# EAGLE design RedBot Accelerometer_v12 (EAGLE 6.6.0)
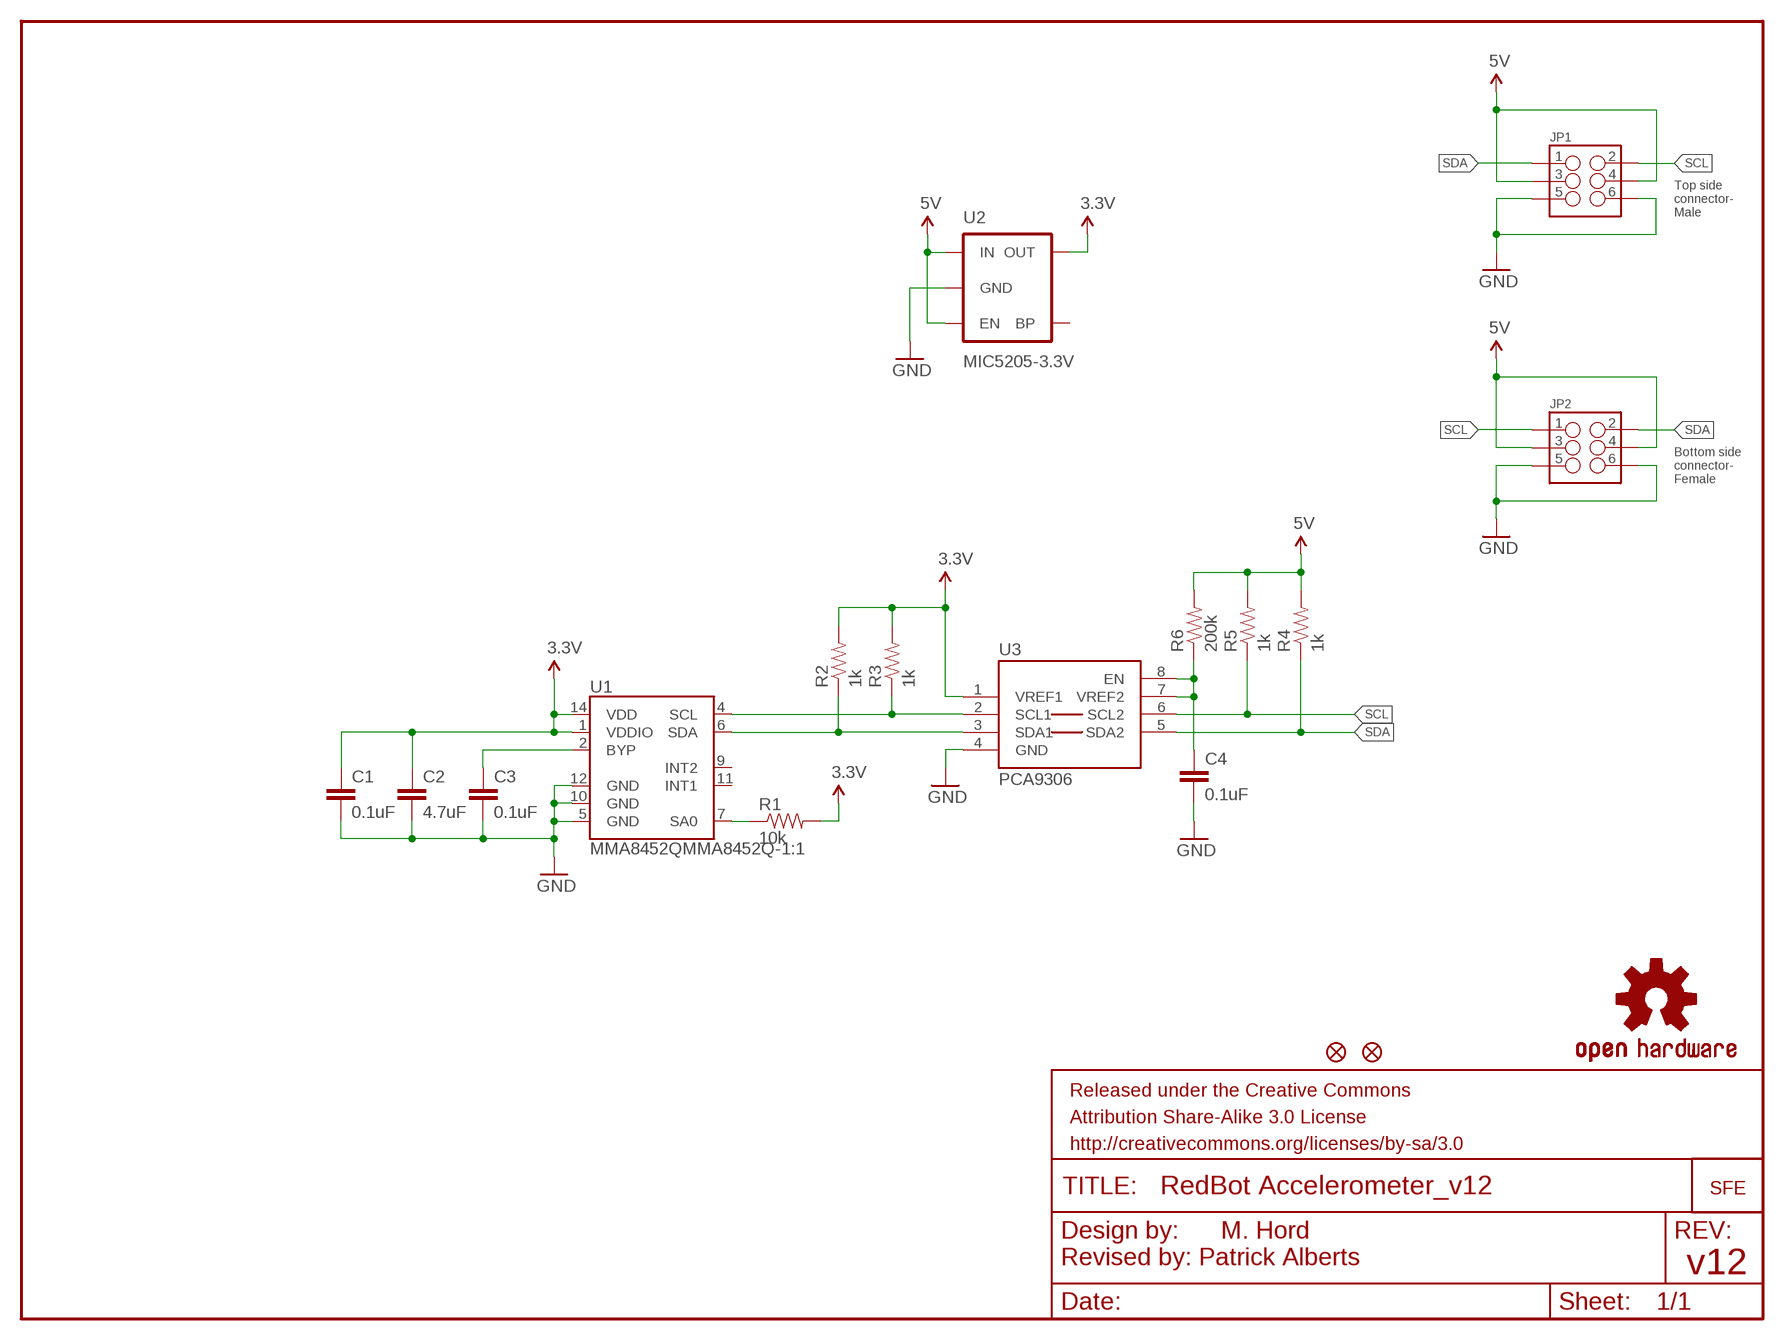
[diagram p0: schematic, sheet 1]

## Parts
C1  0.1uF  0.1UF-25V(+80/-20%)(0603)  [0603-CAP]
C2  4.7uF  4.7UF-6.3V-10%(0603)0603  [0603-CAP]
C3  0.1uF  0.1UF-25V(+80/-20%)(0603)  [0603-CAP]
C4  0.1uF  0.1UF-25V(+80/-20%)(0603)  [0603-CAP]
FID1  FIDUCIAL1X2  [FIDUCIAL-1X2]
FID3  FIDUCIAL1X2  [FIDUCIAL-1X2]
FRAME1  FRAME-LETTER  [CREATIVE_COMMONS]
JP1  M03X2SMT  [2X3_SMT_POSTS]
JP2  M03X2FEMALE_SMD  [2X3_SMD]
LOGO1  LOGO-SFESK  [SFE-LOGO-FLAME]
LOGO2  OSHW-LOGOS  [OSHW-LOGO-S]
R1  10k  10KOHM1/10W1%(0603)0603  [0603-RES]
R2  1k  1K-1%  [0603-RES]
R3  1k  1K-1%  [0603-RES]
R4  1k  1K-1%  [0603-RES]
R5  1k  1K-1%  [0603-RES]
R6  200k  200KOHM1/10W1%(0603)200K  [0603-RES]
U1  MMA8452QMMA8452Q-1:1  [MMA8452Q-1:1]
U2  MIC5205-3.3V  MIC52053.3V  [SOT23-5]
U3  PCA9306  PCA9306PCA9306DC-1:1  [PCA9306DC-1:1]

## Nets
3.3V: C1.1 C2.1 R1.2 R2.2 R3.2 U1.1(VDDIO) U1.14(VDD) U2.5(OUT) U3.1(VREF1)
5V: JP1.3 JP1.4 JP2.3 JP2.4 R4.2 R5.2 R6.2 U2.1(IN) U2.3(EN)
ADDR: R1.1 U1.7(SA0)
GND: C1.2 C2.2 C3.2 C4.2 JP1.5 JP1.6 JP2.5 JP2.6 U1.5(GND) U1.10(GND) U1.12(GND) U2.2(GND) U3.4(GND)
N$1: C3.1 U1.2(BYP)
N$2: C4.1 R6.1 U3.7(VREF2) U3.8(EN)
SCL: JP1.2 JP2.1 R5.1 U3.6(SCL2)
SCL1: R3.1 U1.4(SCL) U3.2(SCL1)
SDA: JP1.1 JP2.2 R4.1 U3.5(SDA2)
SDA1: R2.1 U1.6(SDA) U3.3(SDA1)
Unconnected: U1.9(INT2) U1.11(INT1) U2.4(BP)

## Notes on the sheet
- Top side
  connector-
  Male
- Bottom side
  connector-
  Female
- M. Hord
- Revised by: Patrick Alberts
- v12

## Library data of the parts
C1 C3 C4 = SparkFun-Capacitors:0.1UF-25V(+80/-20%)(0603): Ceramic; PROD_ID: CAP-00810
C2 = SparkFun-Capacitors:4.7UF-6.3V-10%(0603): CAP-08280; PROD_ID: CAP-08280
FID1 FID3 = SparkFun-Aesthetics:FIDUCIAL: Fiducial Alignment Points
FRAME1 = SparkFun-Aesthetics:FRAME-LETTER: Schematic Frame
JP1 = SparkFun-Connectors:M03X2: 2x3 .1" header. Shrouded, with keying- CONN-10681 SMT- CONN-11415 Pogo pins- HW-11044; PROD_ID: CONN-11415
JP2 = SparkFun-Connectors:M03X2: 2x3 .1" header. Shrouded, with keying- CONN-10681 SMT- CONN-11415 Pogo pins- HW-11044; PROD_ID: CONN-11290
LOGO1 = SparkFun-Aesthetics:LOGO-SFE: Spark Fun Electronics PCB Logo
LOGO2 = SparkFun-Aesthetics:OSHW-LOGO: Open Source Hardware Logo This logo indicates the piece of hardware it is found on incorporates a OSHW license and/or adheres to the definition of open source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
R1 = SparkFun-Resistors:10KOHM1/10W1%(0603): RES-00824; PROD_ID: RES-00824; VALUE: 10K
R2-R5 = SparkFun-Resistors:1K-1%: 1k-ohm SMT; PROD_ID: RES-07856
R6 = SparkFun-Resistors:200KOHM1/10W1%(0603): RES-09385; PROD_ID: RES-09385
U1 = SparkFun-Sensors:MMA8452Q: MMA8452Q 3-Axis, 12/8-bit Digital Accelerometer Supply Voltage: 1.6-3.6V Range: +/- 2g, 4g, 8g Interface: I2C, 12-bit and 8-bit ODR: 1.56 Hz - 800 Hz Package: QFN-16 http://cache.freescale.com/files/sensors/doc/data_sheet/MMA8452Q.pdf
U2 = SparkFun-PowerIC:MIC5205: MIC5205 150mA vreg 3.3V - VREG-00822 5V - VREG-00823; PROD_ID: VREG-00822
U3 = SparkFun-DigitalIC:PCA9306: Bidirectional I2C level shifter. NOT compatible with all available part number pinout schemes- DOUBLE CHECK!!!

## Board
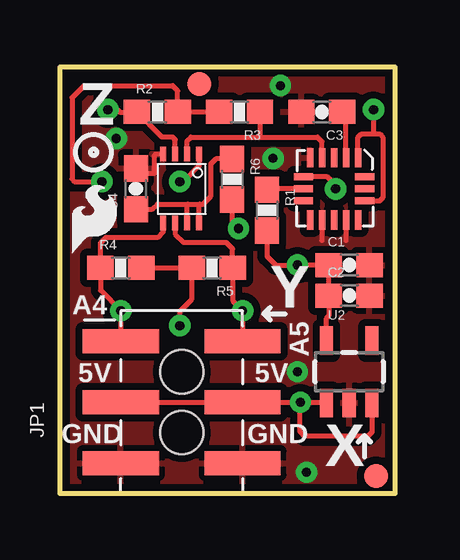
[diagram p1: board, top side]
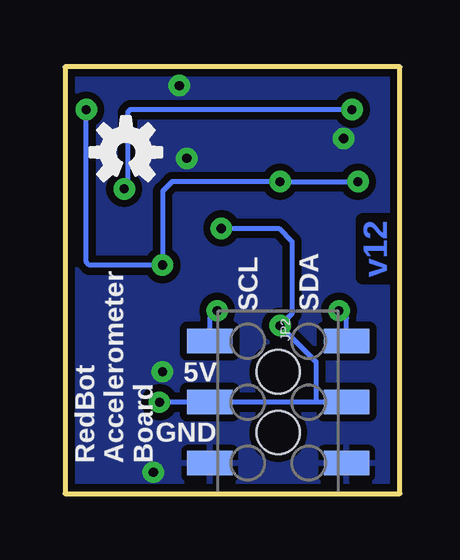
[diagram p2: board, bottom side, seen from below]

Size 13.97 x 17.78 mm. Coordinates in mm from the lower left corner, seen from the top.
Outline: 0,0 0,17.78 13.97,17.78 13.97,0 0,0
Copper layers (1*16): Top 0.035mm / dielectric 1.5mm / Bottom 0.035mm
Design rules "SparkFun-2-layer": minimum track width 7mil, minimum drill 15mil, track to track 8mil, track to pad 8mil, pad to pad 8mil, via to via 8mil, smd to smd 8mil, copper to edge 8mil, drill to drill 8mil, minimum pad ring 12mil, minimum via ring 10mil, stop-mask expansion 4mil, vias tented up to drill 20mil, thermal gap 10mil

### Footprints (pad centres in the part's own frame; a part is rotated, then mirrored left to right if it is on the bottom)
0603-CAP = smd 1.1 x 1: 1 -0.85,0; 2 0.85,0
FIDUCIAL-1X2 = smd 1 x 1: 1 0,0
2X3_SMT_POSTS = smd 1 x 3.17: 1 -2.54,-2.54; 2 -2.54,2.54; 3 0,-2.54; 4 0,2.54; 5 2.54,-2.54; 6 2.54,2.54 | hole 1.8: -1.27,0; 1.27,0
2X3_SMD = smd 1.02 x 1.9: 1 -2.54,-2.85; 2 -2.54,2.85; 3 0,-2.85; 4 0,2.85; 5 2.54,-2.85; 6 2.54,2.85
0603-RES = smd 1.1 x 1: 1 -0.85,0; 2 0.85,0
MMA8452Q-1:1 = smd 0.8 x 0.275: 1 -1.3,1; 2 -1.3,0.5; 3 -1.3,0; 4 -1.3,-0.5; 5 -1.3,-1; 9 1.3,-1; 10 1.3,-0.5; 11 1.3,0; 12 1.3,0.5; 13 1.3,1 | smd 0.29 x 0.8: 6 -0.5,-1.275; 7 0,-1.275; 8 0.5,-1.275; 14 0.5,1.275; 15 0,1.275; 16 -0.5,1.275
SOT23-5 = smd 0.55 x 1.2: 1 -0.95,-1.3; 2 0,-1.3; 3 0.95,-1.3; 4 0.95,1.3; 5 -0.95,1.3
PCA9306DC-1:1 = smd 0.25 x 0.602: 1 -0.73,-1.446; 2 -0.23,-1.446; 3 0.27,-1.446; 4 0.77,-1.446; 5 0.77,1.431; 6 0.27,1.431; 7 -0.23,1.431; 8 -0.73,1.431

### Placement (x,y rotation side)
C1  12.06,9.53 0 top
C2  12.06,8.26 0 top
C3  10.92,15.9 180 top
C4  3.17,12.7 90 top
FID1  5.82,17.07 0 top
FID3  13.18,0.74 0 top
FRAME1  not placed on the board
JP1  5.08,3.81 270 top
JP2  5.08,3.81 270 bottom
LOGO1  0.51,10.03 0 top
LOGO2  11.43,14.22 0 bottom
R1  8.64,11.81 270 top
R2  4.06,15.9 0 top
R3  7.49,15.9 180 top
R4  2.54,9.4 0 top
R5  6.35,9.4 180 top
R6  7.18,13.1 270 top
U1  11.43,12.7 270 top
U2  12.06,5.08 0 top
U3  5.08,12.7 180 top

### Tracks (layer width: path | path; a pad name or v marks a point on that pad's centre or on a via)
3.3V  (via drill 0.38)
  Top 0.203: U2.5 11.12,7.3 11.21,7.41 C2.1 C1.1 v9.91,9.53 9,9.53 8.64,9.89 R1.2 | R3.2 R2.2 4.91,16.79 4.7,17 1,17 0.5,16.5 0.5,13.1 0.6,13 v1.75,13 | U1.1 12.43,14.84 12.57,14.99 13.08,14.99 | 13.08,14.99 13.34,14.99 13.46,14.86 13.46,12.32 13.34,12.2 U1.14 | v13.08,16 13.08,14.99 | v5,13 5.15,13 5.81,13.66 U3.1
  Bottom 0.203: v13.08,16 13.08,9.65 12.95,9.53 v9.91,9.53 v9.9,9.53 9.9,12.6 9.5,13 v5,13 v1.75,13
5V  (via drill 0.38)
  Top 0.203: v10.03,3.81 JP1.4 JP1.3 | v10.03,3.81 11.09,3.81 U2.1 | R4.2 R5.2 5.5,8.1 5,7.6 v5,7 | U2.3 13.02,2.56 12.85,2.4 10.2,2.4 10,2.6 10,3.78 v10.03,3.81 | R6.2 7.18,11.31 v7.45,11.05
  Bottom 0.203: v10.03,3.81 JP2.3 3.5,3.81 | JP2.4 3.5,3.81 | v7.45,11.05 5.05,11.05 4.5,10.5 4.5,7.5 v5,7 3.5,5.5 3.5,3.81
ADDR
  Top 0.203: U1.7 8.68,12.7 R1.1
GND  (via drill 0.38)
  Top 0.203: U1.12 11.93,10.55 11.94,10.54 | U1.10 10.93,10.55 10.92,10.54 | U3.4 3.99,14.15 3.94,14.1 3.94,13.34 3.39,13.34 C4.2
  other vias: 10.29,0.89 9.91,5.08 8.89,13.97 9.2,17 2.35,14.8
  pour Top (isolate 0.305): 0,17.78 13.97,17.78 13.97,0 0,0
  pour Bottom (isolate 0.305): 0,17.78 13.97,17.78 13.97,0 0,0
N$1
  Top 0.203: U1.2 11.93,15.74 C3.1
N$2
  Top 0.203: C4.1 3.85,11.85 4.06,12.06 5.33,12.06 | 5.33,12.06 5.84,12.06 | 5.84,12.06 5.97,12.06 6.3,12.39 6.3,13.75 6.5,13.95 R6.1 | U3.8 5.81,12.03 5.84,12.06 | U3.7 5.31,12.04 5.33,12.06
SCL  (via drill 0.38)
  Top 0.203: U3.6 4.81,10.81 5.15,10.47 6.93,10.47 7.2,10.2 R5.1 7.2,8.04 v7.62,7.62 JP1.2
  Bottom 0.203: JP2.1 7.93,7.31 v7.62,7.62
SCL1
  Top 0.203: U3.2 5.31,14.71 5.46,14.86 8.35,14.86 | 8.35,14.86 10.74,14.86 10.93,14.67 U1.4 | R3.1 8.34,14.87 8.35,14.86
SDA  (via drill 0.38)
  Top 0.203: JP1.1 v2.54,7.62 1.69,8.47 R4.1 1.69,10.45 1.91,10.67 4.06,10.67 4.31,10.91 U3.5
  Bottom 0.203: JP2.2 2.23,7.31 v2.54,7.62
SDA1  (via drill 0.38)
  Top 0.203: v2,16 2.4,16 2.5,15.9 R2.1 4.26,14.86 4.7,14.86 4.81,14.75 U3.3 | v11.5,12.7 11.5,12.85 11.15,13.2 U1.6
  Bottom 0.203: v2,16 11.25,16 11.35,15.9 11.35,12.85 v11.5,12.7

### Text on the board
Bottom: v12
tPlace: Z | Y | A4 | A5 | 5V | 5V | GND | GND | X
bPlace: SDA | SCL | 5V | GND | RedBot / Accelerometer / Board
tDocu: M. Hord | Revised by: Patrick Alberts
